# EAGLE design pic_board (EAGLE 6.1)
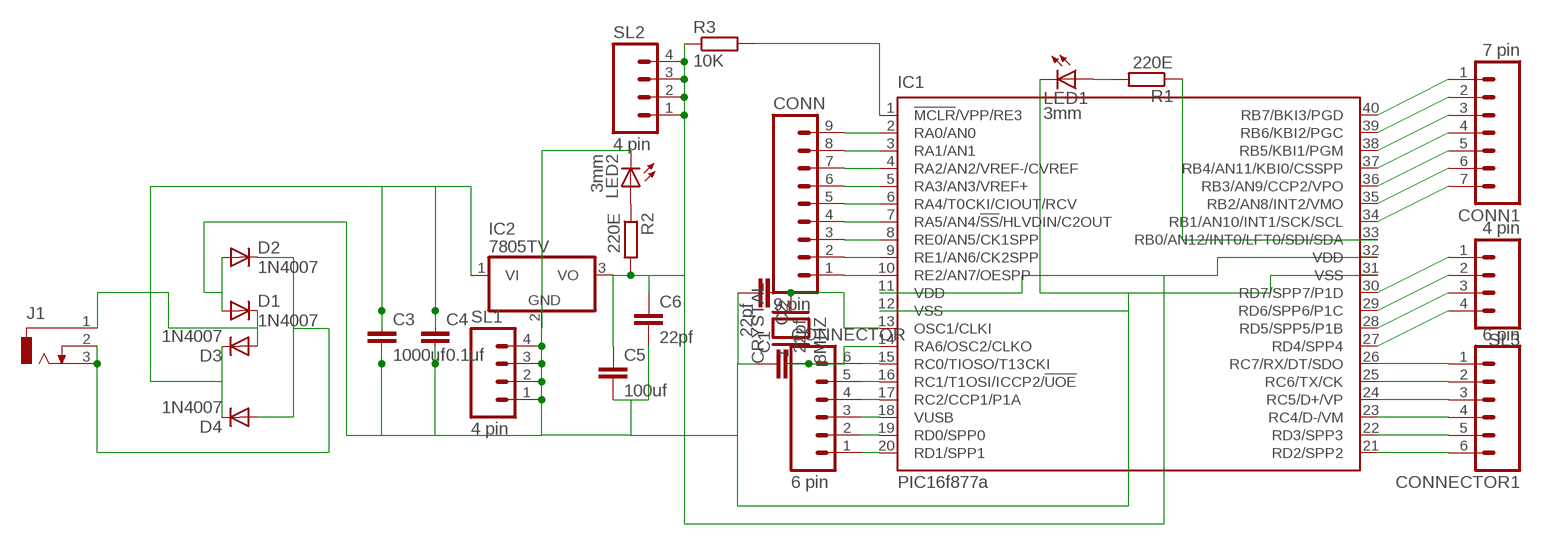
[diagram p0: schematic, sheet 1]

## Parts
C1  22pf  C2.5/2  [C2.5-2]
C2  22pf  C2.5/2  [C2.5-2]
C3  1000uf  C5/7.2  [C5B7.2]
C4  0.1uf  C2,5-3  [C2.5-3]
C5  100uf  C5/7.2  [C5B7.2]
C6  22pf  C2.5/2  [C2.5-2]
CONN  9 pin  M09  [09P]
CONN1  7 pin  M07  [07P]
CONNECTOR  6 pin  M06  [06P]
CONNECTOR1  6 pin  M06  [06P]
CRYSTAL  8MHZ  XTAL/S  [QS]
D1  1N4007  1N4004  [DO41-10]
D2  1N4007  1N4004  [DO41-10]
D3  1N4007  1N4004  [DO41-10]
D4  1N4007  1N4004  [DO41-10]
IC1  PIC16f877a  PIC18F4455_40  [DIL40]
IC2  7805TV  [TO220V]
J1  DCJ0303  [DCJ0303]
LED1  3mm  LED3MM  [LED3MM]
LED2  3mm  LED3MM  [LED3MM]
R1  220E  R-EU_0204/7  [0204/7]
R2  220E  R-EU_0204/7  [0204/7]
R3  10K  R-EU_0204/7  [0204/7]
SL1  4 pin  M04  [04P]
SL2  4 pin  M04  [04P]
SL3  4 pin  M04  [04P]

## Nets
N$1: C2.1 CRYSTAL.2 IC1.13(OSC1/CLKI)
N$2: C1.2 CRYSTAL.1 IC1.14(RA6/OSC2/CLKO)
N$3: LED1.A R1.2
N$4: CONN.1 IC1.10(RE2/AN7/OESPP)
N$5: CONN.2 IC1.9(RE1/AN6/CK2SPP)
N$6: CONN.3 IC1.8(RE0/AN5/CK1SPP)
N$7: CONN.4 IC1.7(RA5/AN4/!SS!/HLVDIN/C2OUT)
N$8: CONN.5 IC1.6(RA4/T0CKI/CIOUT/RCV)
N$9: CONN.6 IC1.5(RA3/AN3/VREF+)
N$10: CONN.7 IC1.4(RA2/AN2/VREF-/CVREF)
N$11: CONN.8 IC1.3(RA1/AN1)
N$12: CONN.9 IC1.2(RA0/AN0)
N$13: CONNECTOR.1 IC1.20(RD1/SPP1)
N$14: CONNECTOR.2 IC1.19(RD0/SPP0)
N$15: CONNECTOR.3 IC1.18(VUSB)
N$16: CONNECTOR.4 IC1.17(RC2/CCP1/P1A)
N$17: CONNECTOR.5 IC1.16(RC1/T1OSI/ICCP2/!UOE)
N$18: CONNECTOR.6 IC1.15(RC0/TIOSO/T13CKI)
N$19: CONN1.1 IC1.40(RB7/BKI3/PGD)
N$20: CONN1.2 IC1.39(RB6/KBI2/PGC)
N$21: CONN1.3 IC1.38(RB5/KBI1/PGM)
N$22: CONN1.4 IC1.37(RB4/AN11/KBI0/CSSPP)
N$23: CONN1.5 IC1.36(RB3/AN9/CCP2/VPO)
N$24: CONN1.6 IC1.35(RB2/AN8/INT2/VMO)
N$25: CONN1.7 IC1.34(RB1/AN10/INT1/SCK/SCL)
N$26: CONNECTOR1.1 IC1.26(RC7/RX/DT/SDO)
N$27: CONNECTOR1.2 IC1.25(RC6/TX/CK)
N$28: CONNECTOR1.3 IC1.24(RC5/D+/VP)
N$29: IC1.33(RB0/AN12/INT0/LFT0/SDI/SDA) R1.1
N$30: C3.1 C4.1 D3.C D4.C IC2.1(VI)
N$31: D2.C D4.A J1.2 J1.3
N$32: D1.C D3.A J1.1
N$33: C5.1 C6.1 IC1.11(VDD) IC1.32(VDD) IC2.3(VO) R2.2 R3.1 SL2.1 SL2.2 SL2.3 SL2.4
N$34: LED2.A R2.1
N$35: C1.1 C2.2 C3.2 C4.2 C5.2 C6.2 D1.A D2.A IC1.12(VSS) IC1.31(VSS) IC2.2(GND) LED1.K(C) LED2.K(C) SL1.1 SL1.2 SL1.3 SL1.4
N$36: CONNECTOR1.4 IC1.23(RC4/D-/VM)
N$37: CONNECTOR1.5 IC1.22(RD3/SPP3)
N$38: CONNECTOR1.6 IC1.21(RD2/SPP2)
N$39: IC1.1(!MCLR!/VPP/RE3) R3.2
N$40: IC1.30(RD7/SPP7/P1D) SL3.1
N$41: IC1.29(RD6/SPP6/P1C) SL3.2
N$42: IC1.28(RD5/SPP5/P1B) SL3.3
N$43: IC1.27(RD4/SPP4) SL3.4

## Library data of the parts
C1-C6 = capacitor-wima:C: CAPACITOR
CONN = con-amp-quick:M09: AMP QUICK CONNECTOR; OC_FARNELL: unknown; OC_NEWARK: unknown
CONN1 = con-amp-quick:M07: AMP QUICK CONNECTOR; OC_FARNELL: unknown; OC_NEWARK: unknown
CONNECTOR CONNECTOR1 = con-amp-quick:M06: AMP QUICK CONNECTOR; OC_FARNELL: unknown; OC_NEWARK: unknown
CRYSTAL = special:XTAL/S: CRYSTAL
D1-D4 = diode:1N4004: DIODE
IC1 = microchip:PIC18F4*_40: USB Microcontrollers with nanoWatt Technology High-Performance, Enhanced Flash, 28/40/44-Pin, Source: http://ww1.microchip.com/downloads/en/devicedoc/39632c.pdf; MF: MICROCHIP; MPN: PIC18F4455-I/P; OC_FARNELL: 9321314; OC_NEWARK: 05K2028
IC2 = linear:78*: Positive VOLTAGE REGULATOR Source: http://cache.national.com/ds/LM/LM78L05.pdf http://www.fairchildsemi.com/ds/LM/LM7805.pdf
J1 = con-jack:DCJ0303: DC POWER JACK Source: DCJ0303.pdf; OC_FARNELL: unknown; OC_NEWARK: unknown
LED1 LED2 = led:LED: LED
R1-R3 = rcl:R-EU_: RESISTOR, European symbol
SL1-SL3 = con-amp-quick:M04: AMP QUICK CONNECTOR; OC_FARNELL: unknown; OC_NEWARK: unknown

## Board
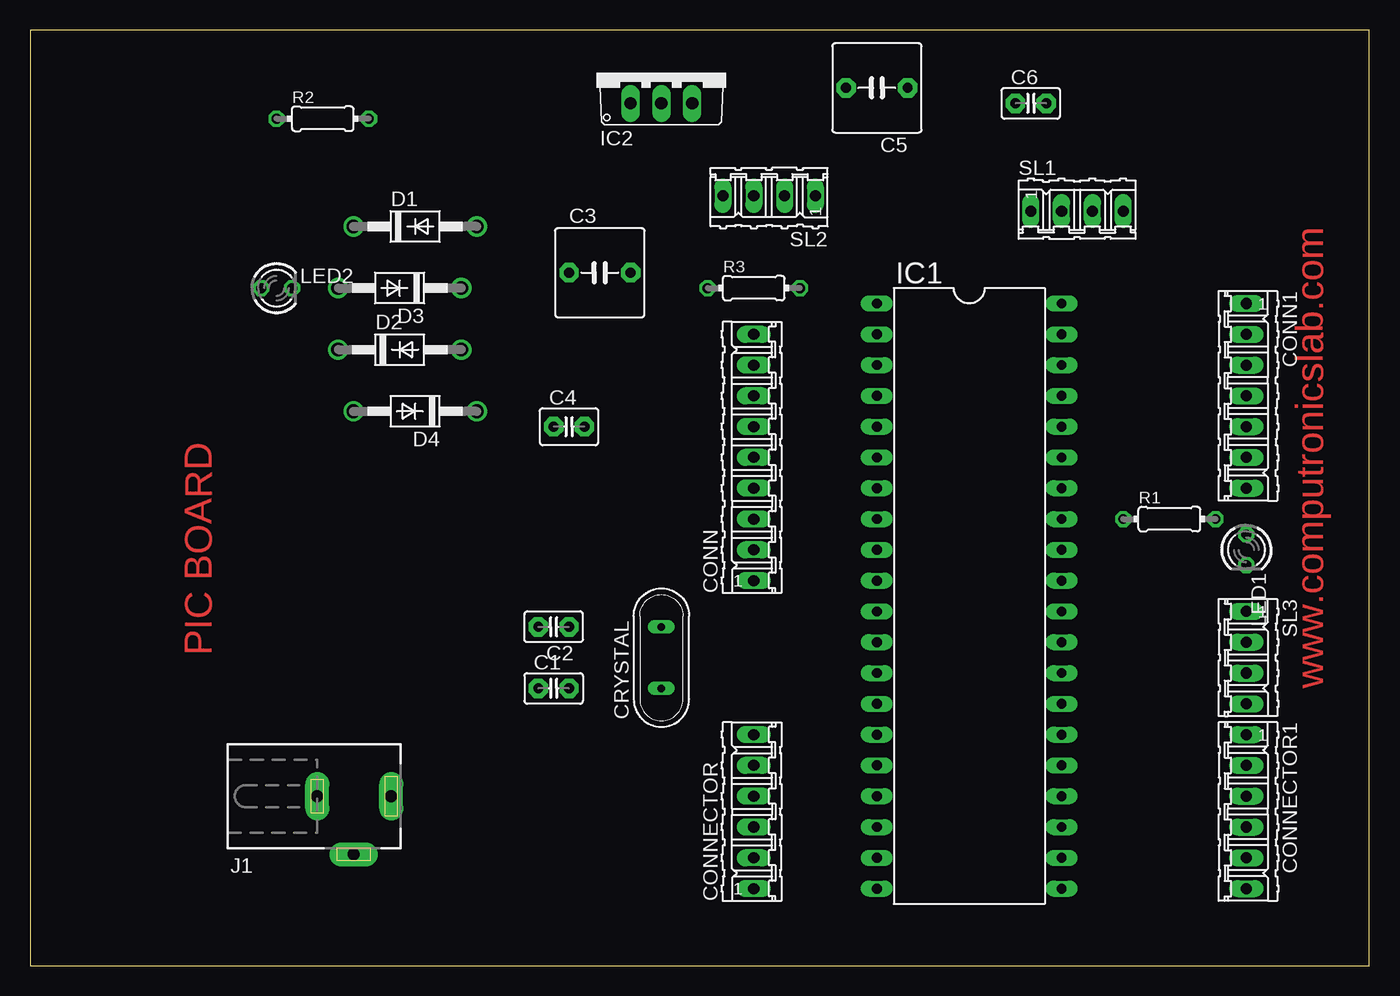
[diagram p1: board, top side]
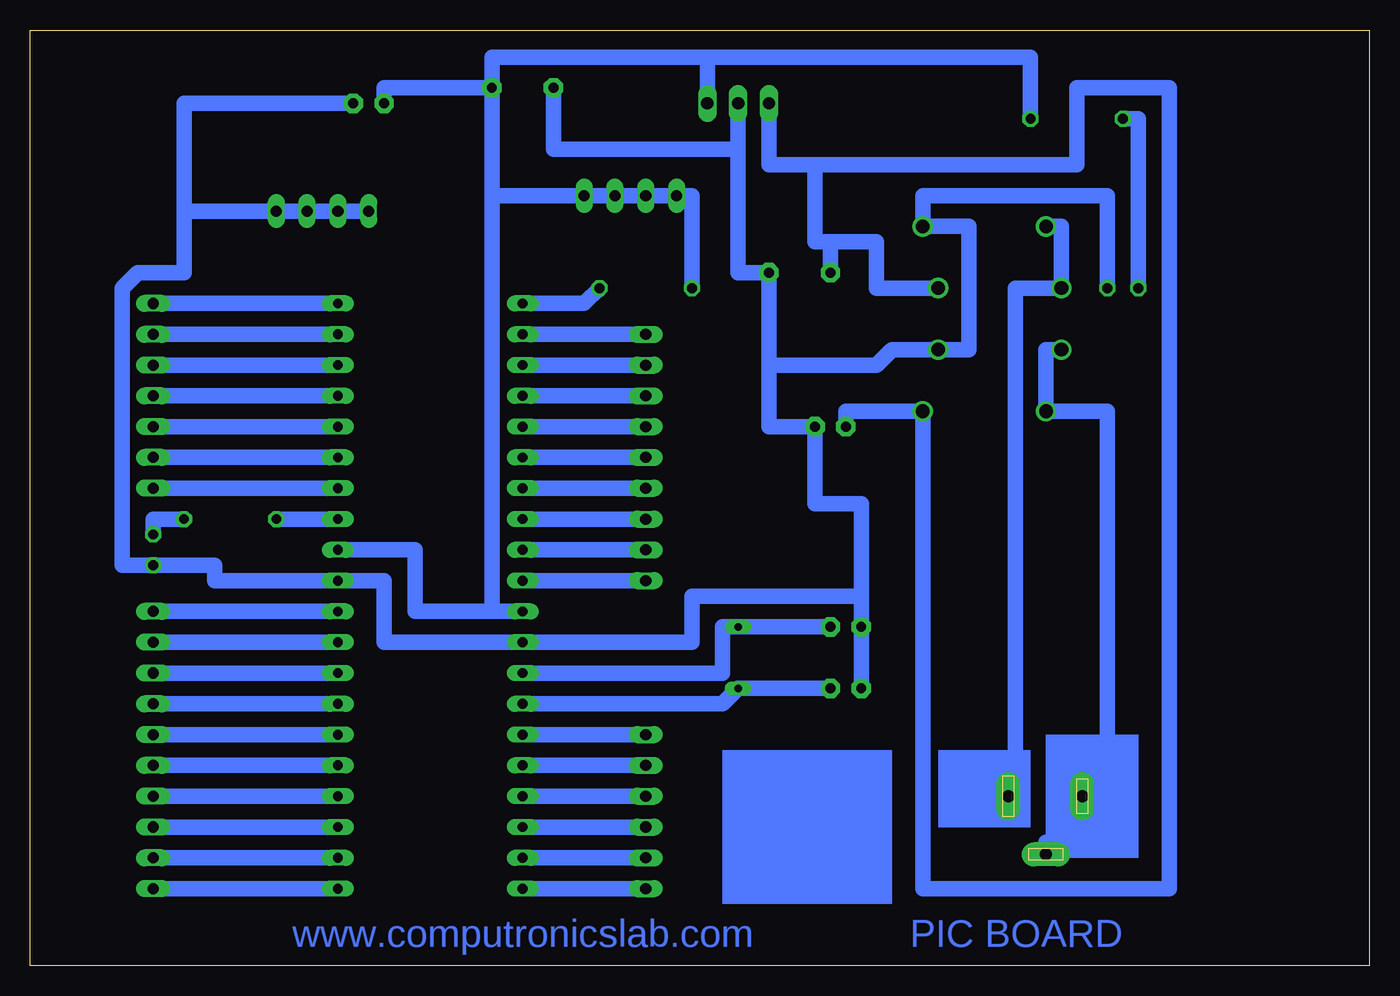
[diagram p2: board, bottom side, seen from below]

Size 110.47 x 77.14 mm. Coordinates in mm from the lower left corner, seen from the top.
Outline: 0,0 110.47,0 110.47,77.14 0,77.14 0,0
Copper layers (1*16): Top 0.035mm / dielectric 1.5mm / Bottom 0.035mm
Design rules: minimum track width 50mil, minimum drill 24mil, track to track 8mil, track to pad 8mil, pad to pad 8mil, via to via 8mil, smd to smd 8mil, copper to edge 40mil, drill to drill 8mil, minimum pad ring 10mil, minimum via ring 8mil, stop-mask expansion 4mil, vias tented up to drill 0mil, thermal gap 10mil

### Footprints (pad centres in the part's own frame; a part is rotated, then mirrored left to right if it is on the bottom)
C2.5-2 = drill 0.813 pad 1.6 octagon: 1 -1.27,0; 2 1.27,0
C5B7.2 = drill 0.813 pad 1.6 octagon: 1 -2.54,0; 2 2.54,0
C2.5-3 = drill 0.813 pad 1.6 octagon: 1 -1.27,0; 2 1.27,0
09P = drill 0.914 long: 1 -10.16,0; 2 -7.62,0; 3 -5.08,0; 4 -2.54,0; 5 0,0; 6 2.54,0; 7 5.08,0; 8 7.62,0; 9 10.16,0
07P = drill 0.914 long: 1 -7.62,0; 2 -5.08,0; 3 -2.54,0; 4 0,0; 5 2.54,0; 6 5.08,0; 7 7.62,0
06P = drill 0.914 long: 1 -6.35,0; 2 -3.81,0; 3 -1.27,0; 4 1.27,0; 5 3.81,0; 6 6.35,0
QS = drill 0.61 long: 1 -2.54,0; 2 2.54,0
DO41-10 = drill 1.118: A 5.08,0; C -5.08,0
DIL40 = drill 0.813 long: 1 -24.13,-7.62; 2 -21.59,-7.62; 3 -19.05,-7.62; 4 -16.51,-7.62; 5 -13.97,-7.62; 6 -11.43,-7.62; 7 -8.89,-7.62; 8 -6.35,-7.62; 9 -3.81,-7.62; 10 -1.27,-7.62; 11 1.27,-7.62; 12 3.81,-7.62; 13 6.35,-7.62; 14 8.89,-7.62; 15 11.43,-7.62; 16 13.97,-7.62; 17 16.51,-7.62; 18 19.05,-7.62; 19 21.59,-7.62; 20 24.13,-7.62; 21 24.13,7.62; 22 21.59,7.62; 23 19.05,7.62; 24 16.51,7.62; 25 13.97,7.62; 26 11.43,7.62; 27 8.89,7.62; 28 6.35,7.62; 29 3.81,7.62; 30 1.27,7.62; 31 -1.27,7.62; 32 -3.81,7.62; 33 -6.35,7.62; 34 -8.89,7.62; 35 -11.43,7.62; 36 -13.97,7.62; 37 -16.51,7.62; 38 -19.05,7.62; 39 -21.59,7.62; 40 -24.13,7.62
TO220V = drill 1.016 long: 1 -2.54,-2.54; 2 0,-2.54; 3 2.54,-2.54
DCJ0303 = drill 1 pad 2 long: 1 0,3.1; 2 4.8,0; 3 0,-3
LED3MM = drill 0.813 octagon: A -1.27,0; K 1.27,0
0204/7 = drill 0.813 octagon: 1 -3.81,0; 2 3.81,0
04P = drill 0.914 long: 1 -3.81,0; 2 -1.27,0; 3 1.27,0; 4 3.81,0

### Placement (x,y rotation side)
C1  43.18,22.86 0 top
C2  43.18,27.94 180 top
C3  46.99,57.15 0 top
C4  44.45,44.45 0 top
C5  69.85,72.39 180 top
C6  82.55,71.12 0 top
CONN  59.69,41.91 90 top
CONN1  100.33,46.99 270 top
CONNECTOR  59.69,12.7 90 top
CONNECTOR1  100.33,12.7 270 top
CRYSTAL  52.07,25.4 90 top
D1  31.75,60.96 0 top
D2  30.48,50.8 0 top
D3  30.48,55.88 180 top
D4  31.75,45.72 180 top
IC1  77.47,30.48 270 top
IC2  52.07,73.66 0 top
J1  26.67,13.97 270 top
LED1  100.33,34.29 270 top
LED2  20.32,55.88 0 top
R1  93.98,36.83 0 top
R2  24.13,69.85 0 top
R3  59.69,55.88 0 top
SL1  86.36,62.23 0 top
SL2  60.96,63.5 180 top
SL3  100.33,25.4 270 top

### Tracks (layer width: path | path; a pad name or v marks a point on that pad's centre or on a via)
N$1
  Bottom 1.27: C2.1 CRYSTAL.2 53.34,27.94 53.34,24.13 IC1.13
N$2
  Bottom 1.27: C1.2 CRYSTAL.1 53.34,21.59 IC1.14
N$3
  Bottom 1.27: LED1.A 100.33,36.83 R1.2
N$4
  Bottom 1.27: CONN.1 IC1.10
N$5
  Bottom 1.27: CONN.2 IC1.9
N$6
  Bottom 1.27: CONN.3 IC1.8
N$7
  Bottom 1.27: CONN.4 IC1.7
N$8
  Bottom 1.27: CONN.5 IC1.6
N$9
  Bottom 1.27: CONN.6 IC1.5
N$10
  Bottom 1.27: CONN.7 IC1.4
N$11
  Bottom 1.27: CONN.8 IC1.3
N$12
  Bottom 1.27: CONN.9 IC1.2
N$13
  Bottom 1.27: CONNECTOR.1 IC1.20
N$14
  Bottom 1.27: CONNECTOR.2 IC1.19
N$15
  Bottom 1.27: CONNECTOR.3 IC1.18
N$16
  Bottom 1.27: CONNECTOR.4 IC1.17
N$17
  Bottom 1.27: CONNECTOR.5 IC1.16
N$18
  Bottom 1.27: CONNECTOR.6 IC1.15
N$19
  Bottom 1.27: CONN1.1 IC1.40
N$20
  Bottom 1.27: CONN1.2 IC1.39
N$21
  Bottom 1.27: CONN1.3 IC1.38
N$22
  Bottom 1.27: CONN1.4 IC1.37
N$23
  Bottom 1.27: CONN1.5 IC1.36
N$24
  Bottom 1.27: CONN1.6 IC1.35
N$25
  Bottom 1.27: CONN1.7 IC1.34
N$26
  Bottom 1.27: CONNECTOR1.1 IC1.26
N$27
  Bottom 1.27: CONNECTOR1.2 IC1.25
N$28
  Bottom 1.27: CONNECTOR1.3 IC1.24
N$29
  Bottom 1.27: R1.1 IC1.33
N$30
  Bottom 1.27: C4.1 43.18,45.72 D4.C 36.83,6.35 16.51,6.35 16.51,72.39 24.13,72.39 24.13,66.04 45.72,66.04 | D3.C 40.64,55.88 40.64,59.69 44.45,59.69 | 44.45,59.69 45.72,59.69 45.72,66.04 | 45.72,66.04 49.53,66.04 IC2.1 | 44.45,59.69 C3.1
N$31
  Bottom 1.27: D2.C 26.67,50.8 D4.A 21.59,45.72 21.59,13.97 | 21.59,13.97 21.59,10.16 26.67,10.16 J1.2 | J1.3 21.59,13.97
N$32
  Bottom 1.27: D1.C 25.4,60.96 D3.A 29.21,55.88 29.21,13.97 J1.1
N$33
  Bottom 1.27: 72.39,29.21 78.74,29.21 78.74,34.29 IC1.32 | 72.39,29.21 IC1.11 | R2.2 27.94,74.93 54.61,74.93 | C5.1 72.39,74.93 54.61,74.93 | 72.39,63.5 C5.1 | 54.61,74.93 IC2.3 | C6.1 81.28,72.39 C5.1 | 72.39,63.5 72.39,29.21 | 72.39,63.5 SL2.1 SL2.2 SL2.3 SL2.4 55.88,63.5 R3.1
N$34
  Bottom 1.27: LED2.A 19.05,69.85 R2.1
N$35
  Bottom 1.27: 97.79,62.23 97.79,57.15 101.6,57.15 102.87,55.88 102.87,33.02 LED1.K 95.25,33.02 95.25,31.75 IC1.31 81.28,31.75 81.28,26.67 IC1.12 55.88,26.67 55.88,30.48 41.91,30.48 | 97.79,62.23 97.79,71.12 C6.2 | 52.07,67.31 52.07,57.15 C3.2 49.53,49.53 | 52.07,67.31 IC2.2 | C5.2 67.31,67.31 52.07,67.31 | LED2.K 21.59,63.5 36.83,63.5 D1.A 33.02,60.96 33.02,50.8 D2.A 39.37,50.8 40.64,49.53 49.53,49.53 | C1.1 C2.2 41.91,30.48 | 49.53,49.53 49.53,44.45 C4.2 45.72,38.1 41.91,38.1 41.91,30.48 | SL1.1 SL1.2 SL1.3 SL1.4 97.79,62.23
N$36
  Bottom 1.27: CONNECTOR1.4 IC1.23
N$37
  Bottom 1.27: CONNECTOR1.5 IC1.22
N$38
  Bottom 1.27: CONNECTOR1.6 IC1.21
N$39
  Bottom 1.27: R3.2 64.77,54.61 IC1.1
N$40
  Bottom 1.27: SL3.1 IC1.30
N$41
  Bottom 1.27: SL3.2 IC1.29
N$42
  Bottom 1.27: SL3.3 IC1.28
N$43
  Bottom 1.27: SL3.4 IC1.27
(copper drawn outside any net)
  shapes: Bottom area x3

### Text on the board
Top: PIC BOARD | www.computronicslab.com
Bottom: PIC BOARD | www.computronicslab.com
